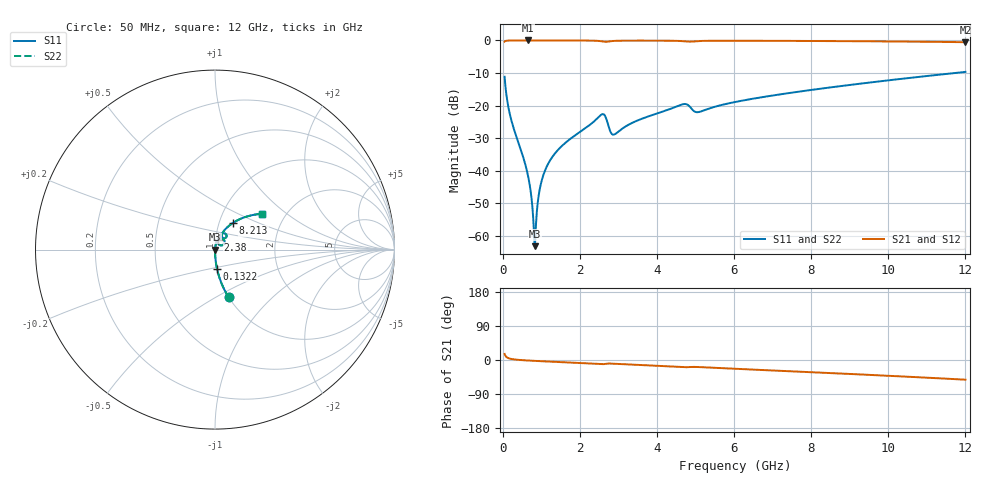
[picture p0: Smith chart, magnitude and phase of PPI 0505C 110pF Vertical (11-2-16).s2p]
# GHz S MA R 50
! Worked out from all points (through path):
!   1601 points, 50 MHz to 12 GHz, reference 50 ohm
!   highest |S21| = -0.01 dB at 655 MHz (marker M1); lowest = -0.5 dB at 12 GHz (marker M2)
!   group delay of S21, straight-line fit = 12.2 ps
!   lowest |S11| = -63.2 dB at 834.2 MHz (marker M3), VSWR 1.00, Z = 50.1 + j0.00818 ohm
!   |S11| at or under -10 dB: start of sweep to 11.73 GHz
!   |S22| runs from -63.2 to -9.7 dB; largest |S21 - S12| = 0
!   S11 on the Smith chart (normalised r, x): 50 MHz: 1.00, -0.57; 132.2 MHz: 1.00, -0.21; 2.38 GHz: 1.03, +0.11; 8.213 GHz: 1.17, +0.36; 12 GHz: 1.52, +0.68
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0.05  0.2764 -74.0  0.9608 15.9  0.9608 15.9  0.2764 -74.0
0.1321563  0.1059 -84.1  0.994 5.7  0.994 5.7  0.1059 -84.1
0.6549687  0.008452 -87.2  0.9993 -1.4  0.9993 -1.4  0.008452 -87.2
0.7296563  0.004641 -83.8  0.9993 -1.8  0.9993 -1.8  0.004641 -83.8
0.796875  0.001641 -68.1  0.9993 -2.2  0.9993 -2.2  0.001641 -68.1
0.8342188  0.0006911 6.8  0.9993 -2.4  0.9993 -2.4  0.0006911 6.8
0.8715625  0.001792 64.6  0.9992 -2.5  0.9992 -2.5  0.001792 64.6
0.9835938  0.006006 79.8  0.9992 -3.1  0.9992 -3.1  0.006006 79.8
1.162844  0.0122 82.2  0.999 -4.0  0.999 -4.0  0.0122 82.2
1.484  0.02233 82.1  0.9987 -5.4  0.9987 -5.4  0.02233 82.1
2.044156  0.04075 79.2  0.9971 -8.1  0.9971 -8.1  0.04075 79.2
2.38025  0.05782 73.0  0.9912 -10.0  0.9912 -10.0  0.05782 73.0
2.61925  0.0733 47.0  0.9589 -10.9  0.9589 -10.9  0.0733 47.0
2.888125  0.03583 53.2  0.9831 -9.9  0.9831 -9.9  0.03583 53.2
4.038312  0.07678 71.4  0.9929 -15.7  0.9929 -15.7  0.07678 71.4
4.688094  0.1051 59.1  0.9727 -19.0  0.9727 -19.0  0.1051 59.1
5.061531  0.07904 56.7  0.9766 -18.5  0.9766 -18.5  0.07904 56.7
6.025  0.1132 64.7  0.9892 -23.3  0.9892 -23.3  0.1132 64.7
8.019156  0.1742 56.8  0.9811 -32.2  0.9811 -32.2  0.1742 56.8
8.213344  0.1804 55.9  0.98 -33.1  0.98 -33.1  0.1804 55.9
10.01331  0.2443 47.5  0.9657 -41.7  0.9657 -41.7  0.2443 47.5
12  0.3284 37.4  0.9399 -51.9  0.9399 -51.9  0.3284 37.4
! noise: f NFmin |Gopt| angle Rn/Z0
0.05  0.000349  0.8501  0.3587  0.0004958
1.372  0.003572  0.643  3.748  0.001891
2.701  0.03496  0.9164  7.568  0.09182
4.031  0.01257  0.694  10.98  0.007939
5.36  0.02089  0.7481  14.73  0.01642
6.682  0.0152  0.6056  17.58  0.00697
8.012  0.01623  0.5696  20.52  0.006613
9.341  0.01801  0.5552  23.43  0.006974
10.67  0.02013  0.5509  26.28  0.007626
12  0.02257  0.5533  29.09  0.008514
